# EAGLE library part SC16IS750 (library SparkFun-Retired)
SPI/I2C/IrDA to UART
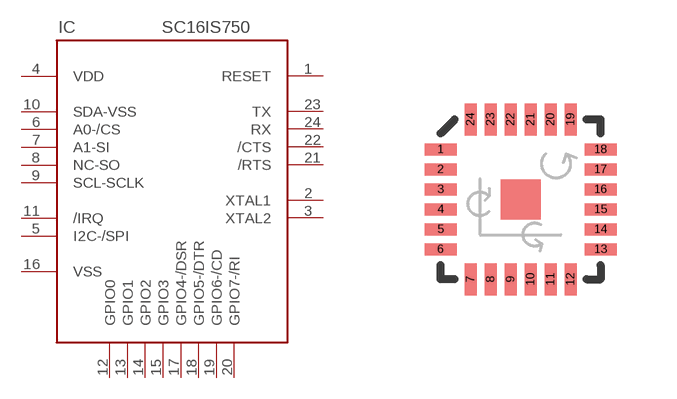
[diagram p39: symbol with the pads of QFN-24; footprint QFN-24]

Designator prefix IC

## SC16IS750  [QFN-24]
1  RESET
2  XTAL1
3  XTAL2
4  VDD
5  I2C-/SPI
6  A0-/CS
7  A1-SI
8  NC-SO
9  SCL-SCLK
10  SDA-VSS
11  /IRQ
12  GPIO0
13  GPIO1
14  GPIO2
15  GPIO3
16  VSS
17  GPIO4-/DSR
18  GPIO5-/DTR
19  GPIO6-/CD
20  GPIO7-/RI
21  /RTS
22  /CTS
23  TX
24  RX

## Footprint QFN-24 (pad centres in mm)
smd 0.8 x 0.3: 1 -2,1.25; 2 -2,0.75; 3 -2,0.25; 4 -2,-0.25; 5 -2,-0.75; 6 -2,-1.25; 13 2,-1.25; 14 2,-0.75; 15 2,-0.25; 16 2,0.25; 17 2,0.75; 18 2,1.25
smd 0.3 x 0.8: 7 -1.25,-2; 8 -0.75,-2; 9 -0.25,-2; 10 0.25,-2; 11 0.75,-2; 12 1.25,-2; 19 1.25,2; 20 0.75,2; 21 0.25,2; 22 -0.25,2; 23 -0.75,2; 24 -1.25,2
